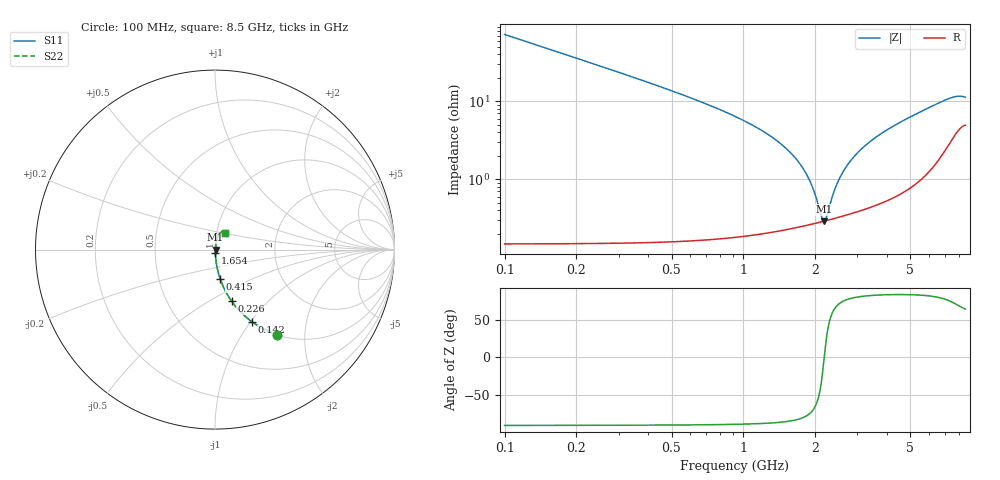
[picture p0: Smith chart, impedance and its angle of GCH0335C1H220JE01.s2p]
!Murata Part Number: GCH0335C1H220JE01
!These Parameters are Measured in Series Mode Connection
!Data Generated on Mar 13, 2026
!  o--ll--o
!Port1  Port2
!  o------o
!Operation Temp=25[degC], DC Bias Voltage=0[V]
!Freq. Start=100[MHz] Stop=9[GHz] 401[Steps]
# Hz S RI R 50
!Freq.(Hz) S11(Real) S11(Imag) S21(Real) S21(Imag) S12(Real) S12(Imag) S22(Real) S22(Imag)
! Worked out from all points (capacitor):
!   401 points, 100 MHz to 8.5 GHz, reference 50 ohm
!   read as one part in series: C = 22 pF near 142 MHz
!   lowest |Z| = 291 mohm at 2.179 GHz (marker M1)
!   series resonance near 2.179 GHz, so ESL is about 240 pH
!   S11 on the Smith chart (normalised r, x): 100 MHz: 1.00, -1.44; 142 MHz: 1.00, -1.01; 226 MHz: 1.00, -0.63; 415 MHz: 1.00, -0.34; 1.654 GHz: 1.00, -0.04; 8.5 GHz: 1.10, +0.20
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1e8  0.3429 -0.4737  0.6571 0.4737  0.6571 0.4737  0.3429 -0.4737
1.42e8  0.2054 -0.4025  0.7946 0.4025  0.7946 0.4025  0.2054 -0.4025
2.26e8  0.0922 -0.287  0.9078 0.287  0.9078 0.287  0.0922 -0.287
4.15e8  0.0288 -0.1628  0.9712 0.1628  0.9712 0.1628  0.0288 -0.1628
7.09e8  0.00986 -0.0901  0.9901 0.0901  0.9901 0.0901  0.00986 -0.0901
1.507e9  0.00287 -0.0248  0.9971 0.0248  0.9971 0.0248  0.00287 -0.0248
1.654e9  0.00272 -0.0183  0.9973 0.0183  0.9973 0.0183  0.00272 -0.0183
1.885e9  0.0027 -0.00955  0.9973 0.00955  0.9973 0.00955  0.0027 -0.00955
1.99e9  0.00274 -0.00597  0.9973 0.00597  0.9973 0.00597  0.00274 -0.00597
2.116e9  0.00284 -0.00193  0.9972 0.00193  0.9972 0.00193  0.00284 -0.00193
2.179e9  0.0029 -8e-06  0.9971 8e-06  0.9971 8e-06  0.0029 -8e-06
2.221e9  0.00295 0.00124  0.9971 -0.00124  0.9971 -0.00124  0.00295 0.00124
2.389e9  0.00316 0.00603  0.9968 -0.00603  0.9968 -0.00603  0.00316 0.00603
2.515e9  0.00335 0.00942  0.9966 -0.00942  0.9966 -0.00942  0.00335 0.00942
2.683e9  0.00364 0.0137  0.9964 -0.0137  0.9964 -0.0137  0.00364 0.0137
2.914e9  0.00409 0.0193  0.9959 -0.0193  0.9959 -0.0193  0.00409 0.0193
3.481e9  0.00548 0.0318  0.9945 -0.0318  0.9945 -0.0318  0.00548 0.0318
4.3e9  0.00822 0.0483  0.9918 -0.0483  0.9918 -0.0483  0.00822 0.0483
5.707e9  0.0163 0.0747  0.9837 -0.0747  0.9837 -0.0747  0.0163 0.0747
7.114e9  0.0346 0.0971  0.9654 -0.0971  0.9654 -0.0971  0.0346 0.0971
7.828e9  0.0489 0.0995  0.9511 -0.0995  0.9511 -0.0995  0.0489 0.0995
8.5e9  0.0561 0.0916  0.9439 -0.0916  0.9439 -0.0916  0.0561 0.0916
